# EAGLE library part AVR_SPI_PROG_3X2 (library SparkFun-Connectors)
AVR ISP 6 Pin This is the reduced ISP connector for AVR programming. Common on Arduino. This footprint will take up less PCB space and can be used with a 10-pin to 6-pin adapter such as SKU: BOB-08508 **Special note about "TEST_POINT" package. The stop mask is on the top side, so if you want your programming test points to be on the bottom of your board, make sure to place this package on the bottom side of the board. This also ensure that the orientation to program from the bottom side will be correct. SparkFun Products: SparkFun ISP Pogo Adapter - NS Tiny AVR Programmer -PTH
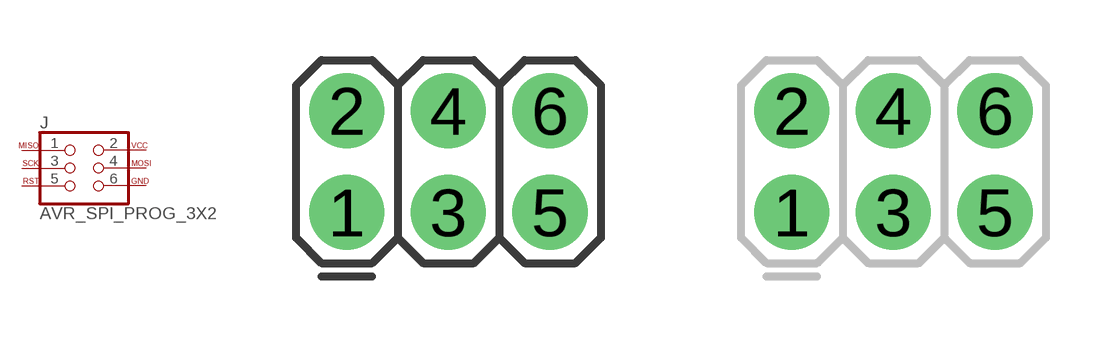
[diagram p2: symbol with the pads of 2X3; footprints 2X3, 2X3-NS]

Designator prefix J

## AVR_SPI_PROG_3X2PTH  [2X3]
1  1  pas
2  2  pas
3  3  pas
4  4  pas
5  5  pas
6  6  pas

## AVR_SPI_PROG_3X2NS  [2X3-NS]
Pads as for 2X3

## AVR_SPI_PROG_3X2OFFSET_PADS  [2X3_OFFSET]
Pads as for 2X3

## AVR_SPI_PROG_3X22X3_LOCK  [2X3_LOCK]
Pads as for 2X3

## AVR_SPI_PROG_3X2TESTPOINTS  [2X3_TEST_POINTS]
Pads as for 2X3

## AVR_SPI_PROG_3X2SMD  [2X3_SMT_POSTS]
Pads as for 2X3

## Footprint 2X3 (pad centres in mm)
Plated Through Hole - 2x3 Specifications: Pin count:6 Pin pitch:0.1" Example device(s): CONN_03x2
drill 1.016 pad 1.88: 1 0,0; 2 0,2.54; 3 2.54,0; 4 2.54,2.54; 5 5.08,0; 6 5.08,2.54

## Footprint 2X3-NS (pad centres in mm)
Plated Through Hole - 2x3 No Silk Outline Specifications: Pin count:6 Pin pitch:0.1" Example device(s): CONN_03x2
drill 1.016 pad 1.88: 1 -2.54,-1.27; 2 -2.54,1.27; 3 0,-1.27; 4 0,1.27; 5 2.54,-1.27; 6 2.54,1.27

## Footprint 2X3_OFFSET (pad centres in mm)
Plated Through Hole - 2x3 Long Pads w/ Offset Holes Specifications: Pin count:6 Pin pitch:0.1" Example device(s): CONN_03x2
drill 1.118 pad 1.88 offset: 1 -2.54,-1.27; 2 -2.54,1.27; 3 0,-1.27; 4 0,1.27; 5 2.54,-1.27; 6 2.54,1.27

## Footprint 2X3_LOCK (pad centres in mm)
Plated Through Hole - 2x3 Locking Footprint Holes are offset from center 0.005", to hold pins in place while soldering. Specifications: Pin count:6 Pin pitch:0.1" Example device(s): CONN_03x2
drill 1.016 pad 1.88: 1 0,0.127; 2 0,2.667; 3 2.54,-0.127; 4 2.54,2.413; 5 5.08,0.127; 6 5.08,2.667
